(* Logix 5000 Rung export; software revision 16.05 *)

MODULES
   Local : vendor None type None code None
   ILX56_PBS : vendor None type None code None
END_MODULES

TYPE PSILX56DPGeneralControl :
STRUCT
   CommandControl : SINT;
   RedundancyControl : SINT;
   DeviceEnable : BOOL[128];   // These bits enable nodes on the PROFIBUS network for data exchange. Each bit represents a node.
END_STRUCT
END_TYPE

TYPE PSILX56DPGeneralStatus :
STRUCT
   ConfigValid : BOOL;
   Owned : BOOL;
   DuplicateDPStation : BOOL;
   ProfibusFieldbusError : BOOL;
   ProfibusDeviceError : BOOL;
   ProfibusOffline : BOOL;
   ProfibusStopped : BOOL;
   ProfibusClear : BOOL;
   ProfibusOperational : BOOL;
   SlaveMode : BOOL;
   ControllerRun : BOOL;
   ModuleRedundancyEnabled : BOOL;
   ModuleRedundancyStatus : BOOL;
   Reserved0 : BOOL;
   Reserved1 : BOOL;
   Reserved2 : BOOL;
   Reserved3 : INT;
   ConfigCRC : INT;
   Reserved4 : DINT;
   DeviceLiveList : BOOL[128];
   DeviceDataExchangeActive : BOOL[128];
   DeviceAlarmPendingFlags : BOOL[128];
   DeviceDiagnosticPendingFlags : BOOL[128];
END_STRUCT
END_TYPE

VAR_GLOBAL   (* controller tags *)
   ILX56PBS_GeneralStatus : PSILX56DPGeneralStatus;
   Local:2:I : AB:1756_MODULE_SINT_500Bytes:I:0;
   Local:2:O : AB:1756_MODULE_SINT_496Bytes:O:0;
   ILX56PBS_GeneralControl : PSILX56DPGeneralControl;
END_VAR

PROGRAM MainProgram

ROUTINE MainRoutine   (* ladder *)
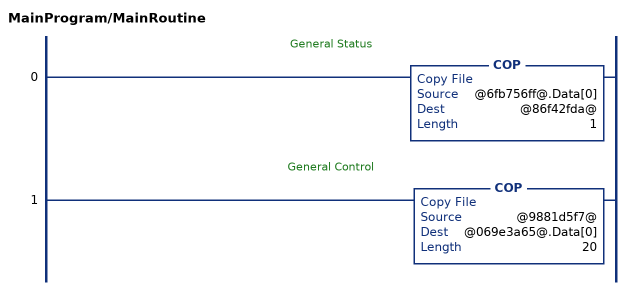
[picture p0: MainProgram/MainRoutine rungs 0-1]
   // General Status
   0: COP(@6fb756ff@.Data[0],@86f42fda@,1);
   // General Control
   1: COP(@9881d5f7@,@069e3a65@.Data[0],20);
END_ROUTINE
END_PROGRAM
